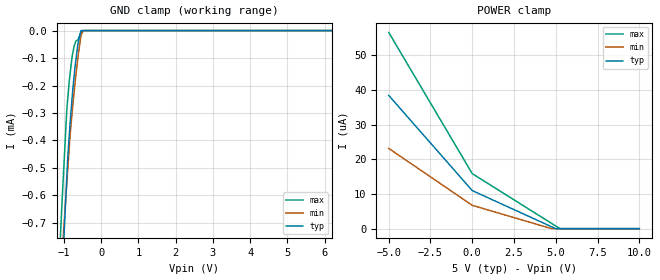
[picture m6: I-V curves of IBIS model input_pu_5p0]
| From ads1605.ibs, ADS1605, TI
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|   INPUT_PU 5.0V Model
[Model]   input_pu_5p0
Model_type   Input
Vinl = 1.5
Vinh = 3.5
|   typ   min   max
|   (nom PVT)   (Fast PVT)   (Slow PVT)
C_comp   3.795e-13   3.735e-13   4.445e-13
|Where nom PVT is NOM Process, 5.0V,39C
|   Fast PVT is Strong Process, 5.25V, -40C
|   Slow PVT is Weak Process, 4.75V, 99C
[Model Spec]
Vinl   1.5   1.425   1.575
Vinh   3.5   3.325   3.675
[Voltage Range]   5   4.75   5.25
|Ambient Temperature   25   85   -40
|Junction Temperature
[Temperature Range]   39   99   -40
[Power Clamp Reference]   5   4.75   5.25
[GND Clamp Reference]   0   0   0
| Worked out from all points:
|   GND clamp passes 1 mA (typ) near -1.09 V on its own axis
[GND Clamp]
|   Voltage   I(typ)   I(min)   I(max)
-5V       -13.49mA   -9.526mA   -14.31mA
-1.091V   -1.007mA   -889.8uA   -734uA
-1.047V   -882.6uA   -801.7uA   -610.5uA
-926mV    -540uA     -559.8uA   -292.3uA
-900mV    -466.2uA   -507.8uA   -249.9uA
-857.8mV  -381.2uA   -423.1uA   -182.9uA
-779mV    -240.7uA   -295.7uA   -93.84uA
-700mV    -127.7uA   -186.9uA   -45.61uA
-620mV    -44.71uA   -92.51uA   -31.58uA
-544.5mV  0A         -19.04uA   -7.919uA
-474.5mV  0A         0A         0A
10V       0A         0A         0A
[POWER Clamp]
|   Voltage   I(typ)   I(min)   I(max)
-5V       38.48uA    23.18uA    56.67uA
3.25mV    10.99uA    6.731uA    15.87uA
4.752V    545.9nA    0A         1.516uA
5V        0A         0A         765.7nA
5.253V    0A         0A         0A
10V       0A         0A         0A
